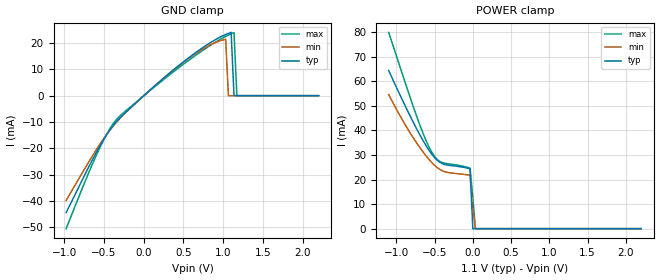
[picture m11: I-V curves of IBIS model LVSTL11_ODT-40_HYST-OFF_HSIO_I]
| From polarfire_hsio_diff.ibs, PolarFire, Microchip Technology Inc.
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|   Model LVSTL11_ODT-40_HYST-OFF_HSIO_I
[Model]   LVSTL11_ODT-40_HYST-OFF_HSIO_I
Model_type   Input
Vinl =   0.083
Vinh =   0.283
|   typ   min   max
C_comp_pullup   1.335e-12   1.335e-12   1.380e-12
C_comp_pulldown  1.335e-12   1.335e-12   1.380e-12
[Temperature Range]  25C   100C   -40C
[Voltage Range]  1.1   1.045   1.155
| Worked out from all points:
|   GND clamp passes 1 mA (typ) near -0.03 V on its own axis
|   POWER clamp passes 1 mA (typ) near -0.00 V on its own axis
[GND Clamp]
| Voltage   I(typ)   I(min)   I(max)
-974.5mV  -44.41mA   -39.8mA    -50.53mA
-577.5mV  -20.6mA    -19.71mA   -21.47mA
-360.9mV  -10.54mA   -10.75mA   -9.764mA
34.38mV   883.4uA    901.9uA    795.5uA
481.3mV   12.39mA    12.3mA     11.52mA
790.6mV   19.21mA    18.56mA    18.15mA
1.031V    23.25mA    21.44mA    22.5mA
1.066V    23.67mA    0A         23.03mA
1.1V      24.04mA    0A         23.52mA
1.136V    0A         0A         23.99mA
1.172V    0A         0A         0A
2.2V      0A         0A         0A
[POWER Clamp]
| Voltage   I(typ)   I(min)   I(max)
-1.1V     64.38mA    54.56mA    79.86mA
-902.3mV  51.16mA    43.27mA    61.19mA
-721.9mV  39.9mA     34.33mA    44.69mA
-613.6mV  33.9mA     29.71mA    36.02mA
-541.4mV  30.51mA    27.07mA    31.39mA
-469.2mV  27.93mA    24.95mA    28.26mA
-397mV    26.42mA    23.53mA    26.84mA
-324.8mV  25.84mA    22.85mA    26.39mA
-36.09mV  24.38mA    21.74mA    24.61mA
0V        0A         8.663mA    12.79mA
34.38mV   0A         0A         0A
2.2V      0A         0A         0A
